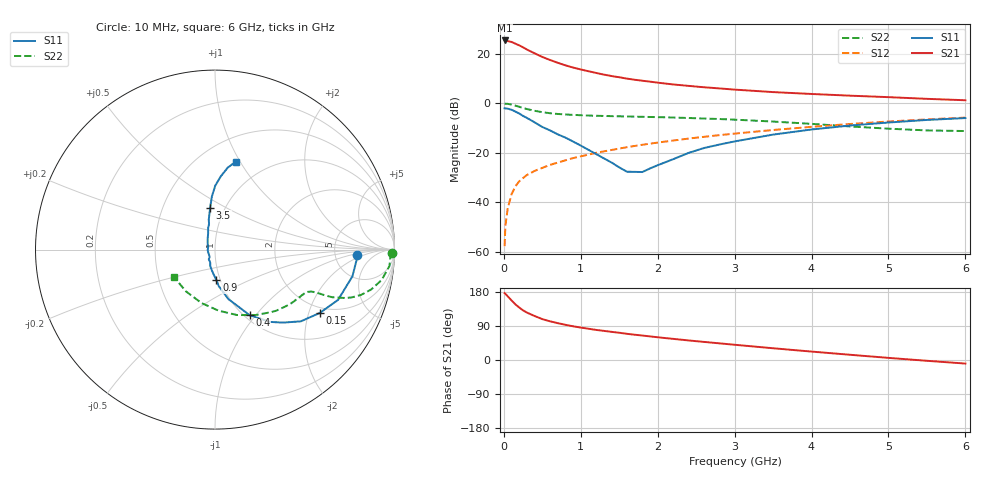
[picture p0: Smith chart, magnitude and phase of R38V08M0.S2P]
! SIEMENS Small Signal Semiconductors
! BFR181
! Si NPN RF Bipolar Junction Transistor in SOT23
! VCE = 8 V  IC = 8 mA
! Common Emitter S-Parameters:  May  1996
# GHz  S  MA  R  50
!  f  S11  S21  S12  S22
! GHz  MAG  ANG  MAG  ANG  MAG  ANG  MAG  ANG
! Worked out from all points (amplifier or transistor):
!   36 points, 10 MHz to 6 GHz, reference 50 ohm
!   highest |S21| = 25.4 dB at 10 MHz (marker M1)
!   |S21| within 3 dB of that: start of sweep to 262 MHz
!   unconditionally stable (mu >= 1): 968.1 MHz to 2.892 GHz
!   at 250 MHz: K = 0.52, MSG = 26.4 dB, |S12| = -30.2 dB
!   at 1.4 GHz: K = 1.04, MAG = 13.6 dB, |S12| = -18.9 dB
!   at 6 GHz: K = 0.86, MSG = 3.5 dB, |S12| = -5.8 dB
!   S11 on the Smith chart (normalised r, x): 10 MHz: 8.44, -1.38; 150 MHz: 1.79, -2.37; 400 MHz: 1.06, -0.93; 900 MHz: 0.96, -0.33; 3.5 GHz: 0.85, +0.42; 6 GHz: 0.73, +0.96
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0.01  0.7931 -2.2  18.61 176.6  0.0013 93.9  0.9876 -1.0
0.02  0.7904 -4.4  18.24 174.5  0.0033 83.0  0.9788 -2.2
0.05  0.78 -11.0  18.08 168.1  0.0075 86.5  0.9762 -5.4
0.1  0.7408 -22.2  17.36 157.3  0.0145 78.8  0.9433 -10.4
0.15  0.682 -31.2  16.02 146.9  0.021 74.0  0.8973 -14.4
0.2  0.6231 -39.9  14.83 138.5  0.0265 71.9  0.8507 -17.3
0.25  0.5562 -47.0  13.5 131.0  0.0309 69.6  0.8043 -19.4
0.3  0.5065 -52.7  12.21 125.1  0.0356 69.0  0.7654 -20.6
0.4  0.4129 -62.2  10.23 116.1  0.0431 67.9  0.7059 -22.1
0.5  0.3326 -68.8  8.641 107.9  0.0496 67.0  0.6617 -22.6
0.6  0.284 -75.1  7.503 102.1  0.057 67.5  0.6306 -22.8
0.7  0.2362 -79.7  6.594 97.3  0.0634 67.5  0.6094 -23.1
0.9  0.169 -87.5  5.279 89.0  0.0781 67.7  0.5844 -23.6
1.1  0.1148 -99.3  4.444 82.5  0.0921 68.0  0.5663 -24.6
1.3  0.0773 -110.0  3.802 76.9  0.107 67.7  0.5549 -26.1
1.6  0.0415 -149.3  3.155 69.1  0.1299 66.7  0.5424 -28.9
1.8  0.0409 158.0  2.86 64.6  0.1453 66.0  0.5335 -31.1
2.2  0.0741 123.4  2.406 55.8  0.177 63.9  0.5161 -36.1
3.5  0.2333 96.7  1.685 31.0  0.2888 53.7  0.428 -58.5
4.5  0.3559 89.8  1.427 13.8  0.3821 43.2  0.341 -86.6
5.5  0.4616 81.2  1.231 -2.1  0.4731 31.0  0.2835 -124.7
6  0.5036 76.7  1.153 -9.4  0.5145 24.2  0.2752 -146.4
